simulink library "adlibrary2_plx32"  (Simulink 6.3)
undefined symbols (not defined in the file or in its folder): clock_ratio, program
libraries: xbsIndex_r4 x36, adlibrary2_plx32 x1

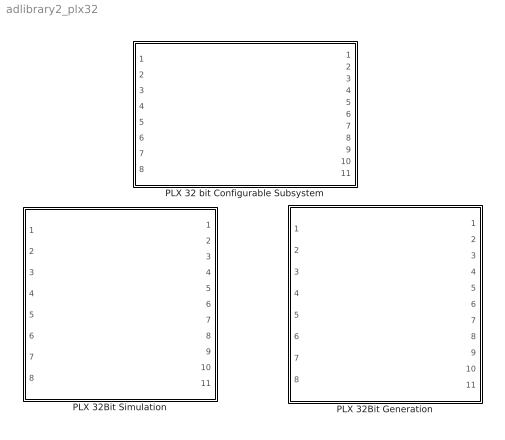
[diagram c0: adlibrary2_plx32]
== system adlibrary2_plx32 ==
  PLX 32 bit Configurable Subsystem : Subsystem  Tag=configX  BlockChoice=PLX 32Bit Simulation  mask{program=program, clock_ratio=clock_ratio}
      mask prompts: program "Local Bus Script Program"; clock_ratio "Clock Ratio"
  PLX 32Bit Generation : Subsystem
  PLX 32Bit Simulation : Subsystem  mask{program=program, clock_ratio=clock_ratio}
      mask prompts: program "Local Bus Script Program"; clock_ratio "Clock Ratio"

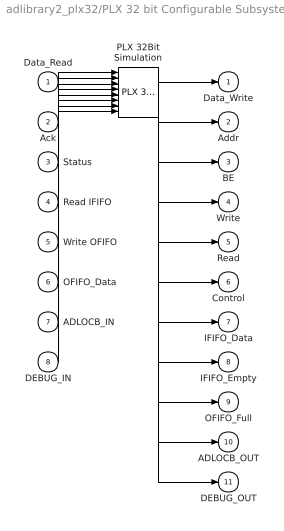
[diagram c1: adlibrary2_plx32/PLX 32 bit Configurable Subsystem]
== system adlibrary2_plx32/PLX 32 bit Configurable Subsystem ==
  Data_Read : Inport
  Ack : Inport  Port=2
  Status : Inport  Port=3
  Read IFIFO : Inport  Port=4
  Write OFIFO : Inport  Port=5
  OFIFO_Data : Inport  Port=6
  ADLOCB_IN : Inport  Port=7
  DEBUG_IN : Inport  Port=8
  PLX 32Bit Simulation : adlibrary2_plx32/PLX 32Bit Simulation  program=program  clock_ratio=clock_ratio
  Data_Write : Outport
  Addr : Outport  Port=2
  BE : Outport  Port=3
  Write : Outport  Port=4
  Read : Outport  Port=5
  Control : Outport  Port=6
  IFIFO_Data : Outport  Port=7
  IFIFO_Empty : Outport  Port=8
  OFIFO_Full : Outport  Port=9
  ADLOCB_OUT : Outport  Port=10
  DEBUG_OUT : Outport  Port=11
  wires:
  Data_Read/1 -> PLX 32Bit Simulation/1
  Ack/1 -> PLX 32Bit Simulation/2
  Status/1 -> PLX 32Bit Simulation/3
  Read IFIFO/1 -> PLX 32Bit Simulation/4
  Write OFIFO/1 -> PLX 32Bit Simulation/5
  OFIFO_Data/1 -> PLX 32Bit Simulation/6
  ADLOCB_IN/1 -> PLX 32Bit Simulation/7
  DEBUG_IN/1 -> PLX 32Bit Simulation/8
  PLX 32Bit Simulation/1 -> Data_Write/1
  PLX 32Bit Simulation/2 -> Addr/1
  PLX 32Bit Simulation/3 -> BE/1
  PLX 32Bit Simulation/4 -> Write/1
  PLX 32Bit Simulation/5 -> Read/1
  PLX 32Bit Simulation/6 -> Control/1
  PLX 32Bit Simulation/7 -> IFIFO_Data/1
  PLX 32Bit Simulation/8 -> IFIFO_Empty/1
  PLX 32Bit Simulation/9 -> OFIFO_Full/1
  PLX 32Bit Simulation/10 -> ADLOCB_OUT/1
  PLX 32Bit Simulation/11 -> DEBUG_OUT/1

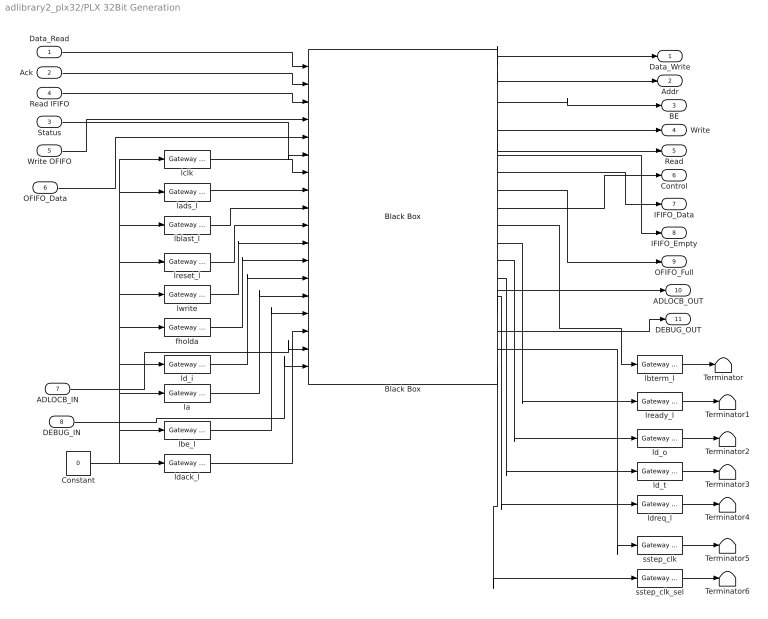
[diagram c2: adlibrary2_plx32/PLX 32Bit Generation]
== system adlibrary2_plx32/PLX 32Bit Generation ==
  Data_Read : Inport
  Ack : Inport  Port=2
  Status : Inport  Port=3
  Read IFIFO : Inport  Port=4
  Write OFIFO : Inport  Port=5
  OFIFO_Data : Inport  Port=6
  ADLOCB_IN : Inport  Port=7
  DEBUG_IN : Inport  Port=8
  Black Box : xbsIndex_r4/Black Box  init_code=lbif32_plx_config  sim_method=Inactive  block_type=blackbox2
  Constant : Constant  Value=0
  Terminator{,1..6} (7 alike) : Terminator
  fholda : xbsIndex_r4/Gateway In  arith_type=Boolean  n_bits=8  bin_pt=6  period=1  dbl_ovrd=off  timing_constraint=None  locs_specified=off  LOCs={}  block_type=gatewayin
  la : xbsIndex_r4/Gateway In  arith_type=Unsigned  n_bits=24  bin_pt=0  period=1  dbl_ovrd=off  timing_constraint=None  locs_specified=off  LOCs={}  block_type=gatewayin
  lads_l : xbsIndex_r4/Gateway In  arith_type=Boolean  n_bits=8  bin_pt=6  period=1  dbl_ovrd=off  timing_constraint=None  locs_specified=off  LOCs={}  block_type=gatewayin
  lbe_l : xbsIndex_r4/Gateway In  arith_type=Unsigned  n_bits=4  bin_pt=0  period=1  dbl_ovrd=off  timing_constraint=None  locs_specified=off  LOCs={}  block_type=gatewayin
  lblast_l : xbsIndex_r4/Gateway In  arith_type=Boolean  n_bits=8  bin_pt=6  period=1  dbl_ovrd=off  timing_constraint=None  locs_specified=off  LOCs={}  block_type=gatewayin
  lbterm_l : xbsIndex_r4/Gateway Out  hdl_port=on  timing_constraint=None  locs_specified=off  LOCs={}  block_type=gatewayout
  lclk : xbsIndex_r4/Gateway In  arith_type=Boolean  n_bits=8  bin_pt=6  period=1  dbl_ovrd=off  timing_constraint=None  locs_specified=off  LOCs={}  block_type=gatewayin
  ld_i : xbsIndex_r4/Gateway In  arith_type=Unsigned  n_bits=32  bin_pt=0  period=1  dbl_ovrd=off  timing_constraint=None  locs_specified=off  LOCs={}  block_type=gatewayin
  ld_o : xbsIndex_r4/Gateway Out  hdl_port=on  timing_constraint=None  locs_specified=off  LOCs={}  block_type=gatewayout
  ld_t : xbsIndex_r4/Gateway Out  hdl_port=on  timing_constraint=None  locs_specified=off  LOCs={}  block_type=gatewayout
  ldack_l : xbsIndex_r4/Gateway In  arith_type=Unsigned  n_bits=2  bin_pt=0  period=1  dbl_ovrd=off  timing_constraint=None  locs_specified=off  LOCs={}  block_type=gatewayin
  ldreq_l : xbsIndex_r4/Gateway Out  hdl_port=on  timing_constraint=None  locs_specified=off  LOCs={}  block_type=gatewayout
  lready_l : xbsIndex_r4/Gateway Out  hdl_port=on  timing_constraint=None  locs_specified=off  LOCs={}  block_type=gatewayout
  lreset_l : xbsIndex_r4/Gateway In  arith_type=Boolean  n_bits=8  bin_pt=6  period=1  dbl_ovrd=off  timing_constraint=None  locs_specified=off  LOCs={}  block_type=gatewayin
  lwrite : xbsIndex_r4/Gateway In  arith_type=Boolean  n_bits=8  bin_pt=6  period=1  dbl_ovrd=off  timing_constraint=None  locs_specified=off  LOCs={}  block_type=gatewayin
  sstep_clk : xbsIndex_r4/Gateway Out  hdl_port=on  timing_constraint=None  locs_specified=off  LOCs={}  block_type=gatewayout
  sstep_clk_sel : xbsIndex_r4/Gateway Out  hdl_port=on  timing_constraint=None  locs_specified=off  LOCs={}  block_type=gatewayout
  Data_Write : Outport
  Addr : Outport  Port=2
  BE : Outport  Port=3
  Write : Outport  Port=4
  Read : Outport  Port=5
  Control : Outport  Port=6
  IFIFO_Data : Outport  Port=7
  IFIFO_Empty : Outport  Port=8
  OFIFO_Full : Outport  Port=9
  ADLOCB_OUT : Outport  Port=10
  DEBUG_OUT : Outport  Port=11
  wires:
  Data_Read/1 -> Black Box/1
  Write OFIFO/1 -> Black Box/4
  OFIFO_Data/1 -> Black Box/5
  lclk/1 -> Black Box/7
  lblast_l/1 -> Black Box/9
  lreset_l/1 -> Black Box/10
  lwrite/1 -> Black Box/11
  fholda/1 -> Black Box/12
  ld_i/1 -> Black Box/13
  la/1 -> Black Box/14
  lbe_l/1 -> Black Box/15
  ldack_l/1 -> Black Box/16
  Constant/1 -> ldack_l/1, lclk/1, lads_l/1, lblast_l/1, lreset_l/1, lwrite/1, fholda/1, ld_i/1, la/1, lbe_l/1
  lbterm_l/1 -> Terminator/1
  lready_l/1 -> Terminator1/1
  ld_o/1 -> Terminator2/1
  ld_t/1 -> Terminator3/1
  ldreq_l/1 -> Terminator4/1
  Black Box/1 -> Data_Write/1
  Black Box/2 -> Addr/1
  Black Box/3 -> BE/1
  Black Box/4 -> Write/1
  Black Box/5 -> Read/1
  Black Box/7 -> IFIFO_Data/1
  Black Box/8 -> OFIFO_Full/1
  Black Box/6 -> IFIFO_Empty/1
  Black Box/9 -> Control/1
  Black Box/10 -> lbterm_l/1
  Black Box/11 -> lready_l/1
  Black Box/12 -> ld_o/1
  Black Box/13 -> ld_t/1
  Black Box/14 -> ldreq_l/1
  Ack/1 -> Black Box/2
  Read IFIFO/1 -> Black Box/3
  lads_l/1 -> Black Box/8
  Status/1 -> Black Box/6
  ADLOCB_IN/1 -> Black Box/17
  Black Box/15 -> ADLOCB_OUT/1
  sstep_clk/1 -> Terminator5/1
  sstep_clk_sel/1 -> Terminator6/1
  Black Box/17 -> sstep_clk/1
  Black Box/18 -> sstep_clk_sel/1
  Black Box/16 -> DEBUG_OUT/1
  DEBUG_IN/1 -> Black Box/18

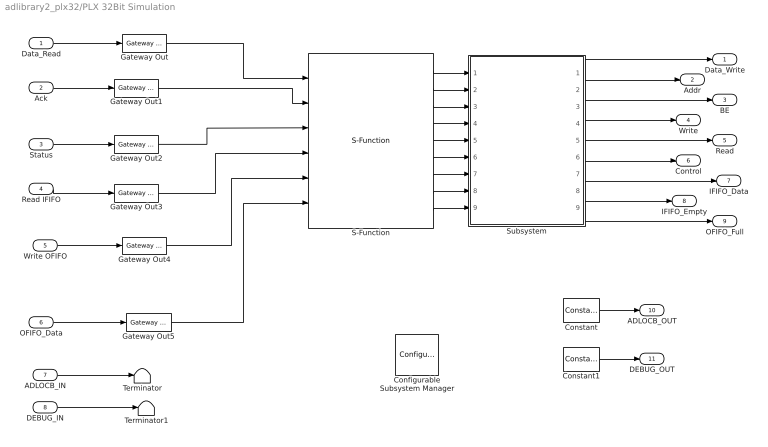
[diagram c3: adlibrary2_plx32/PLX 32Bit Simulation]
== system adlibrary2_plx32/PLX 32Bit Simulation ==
  Data_Read : Inport
  Ack : Inport  Port=2
  Status : Inport  Port=3
  Read IFIFO : Inport  Port=4
  Write OFIFO : Inport  Port=5
  OFIFO_Data : Inport  Port=6
  ADLOCB_IN : Inport  Port=7
  DEBUG_IN : Inport  Port=8
  Configurable Subsystem Manager : xbsIndex_r4/Configurable Subsystem Manager  Tag=xcfgMgr  block_type=configsubsys
  Constant : xbsIndex_r4/Constant  arith_type=Unsigned  const=0  n_bits=34  bin_pt=0  explicit_period=on  period=1  equ=P=C  opselect=C  inp2=PCIN>>17  opr=+  inp1=P  carry=CIN  dbl_ovrd=off  block_type=constant
  Constant1 : xbsIndex_r4/Constant  arith_type=Unsigned  const=0  n_bits=40  bin_pt=0  explicit_period=on  period=1  equ=P=C  opselect=C  inp2=PCIN>>17  opr=+  inp1=P  carry=CIN  dbl_ovrd=off  block_type=constant
  Gateway Out{,1..5} (6 alike) : xbsIndex_r4/Gateway Out  hdl_port=off  timing_constraint=None  locs_specified=off  LOCs={}  block_type=gatewayout
  S-Function : S-Function  FunctionName=lbif_plx32  Parameters=program,clock_ratio
  Subsystem : Subsystem
  Terminator : Terminator
  Terminator1 : Terminator
  Data_Write : Outport
  Addr : Outport  Port=2
  BE : Outport  Port=3
  Write : Outport  Port=4
  Read : Outport  Port=5
  Control : Outport  Port=6
  IFIFO_Data : Outport  Port=7
  IFIFO_Empty : Outport  Port=8
  OFIFO_Full : Outport  Port=9
  ADLOCB_OUT : Outport  Port=10
  DEBUG_OUT : Outport  Port=11
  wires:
  Subsystem/2(Out2) -> Addr/1
  Subsystem/1(Out1) -> Data_Write/1
  S-Function/2 -> Subsystem/2(In2)
  S-Function/1 -> Subsystem/1(In1)
  Gateway Out5/1 -> S-Function/6
  Gateway Out4/1 -> S-Function/5
  Gateway Out3/1 -> S-Function/4
  Gateway Out2/1 -> S-Function/3
  Gateway Out1/1 -> S-Function/2
  Gateway Out/1 -> S-Function/1
  OFIFO_Data/1 -> Gateway Out5/1
  Write OFIFO/1 -> Gateway Out4/1
  Read IFIFO/1 -> Gateway Out3/1
  Status/1 -> Gateway Out2/1
  Ack/1 -> Gateway Out1/1
  Data_Read/1 -> Gateway Out/1
  S-Function/3 -> Subsystem/3(In9)
  Subsystem/3(Out9) -> BE/1
  S-Function/4 -> Subsystem/4(In3)
  S-Function/5 -> Subsystem/5(In4)
  S-Function/6 -> Subsystem/6(In5)
  S-Function/7 -> Subsystem/7(In6)
  S-Function/8 -> Subsystem/8(In7)
  S-Function/9 -> Subsystem/9(In8)
  Subsystem/4(Out3) -> Write/1
  Subsystem/5(Out4) -> Read/1
  Subsystem/6(Out5) -> Control/1
  Subsystem/7(Out6) -> IFIFO_Data/1
  Subsystem/8(Out7) -> IFIFO_Empty/1
  Subsystem/9(Out8) -> OFIFO_Full/1
  ADLOCB_IN/1 -> Terminator/1
  Constant/1 -> ADLOCB_OUT/1
  DEBUG_IN/1 -> Terminator1/1
  Constant1/1 -> DEBUG_OUT/1

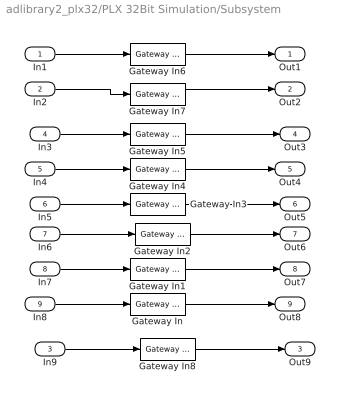
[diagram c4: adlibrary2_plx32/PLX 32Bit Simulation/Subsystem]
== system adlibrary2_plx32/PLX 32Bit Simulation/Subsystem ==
  In1 : Inport
  In2 : Inport  Port=2
  In9 : Inport  Port=3
  In3 : Inport  Port=4
  In4 : Inport  Port=5
  In5 : Inport  Port=6
  In6 : Inport  Port=7
  In7 : Inport  Port=8
  In8 : Inport  Port=9
  Gateway In{,1,4..5} (4 alike) : xbsIndex_r4/Gateway In  arith_type=Boolean  n_bits=8  bin_pt=6  period=1  dbl_ovrd=off  timing_constraint=None  locs_specified=off  LOCs={}  block_type=gatewayin
  Gateway In2 : xbsIndex_r4/Gateway In  arith_type=Unsigned  n_bits=32  bin_pt=0  period=1  dbl_ovrd=off  timing_constraint=None  locs_specified=off  LOCs={}  block_type=gatewayin
  Gateway In3 : xbsIndex_r4/Gateway In  arith_type=Unsigned  n_bits=32  bin_pt=0  period=1  dbl_ovrd=off  timing_constraint=None  locs_specified=off  LOCs={}  block_type=gatewayin
  Gateway In6 : xbsIndex_r4/Gateway In  arith_type=Unsigned  n_bits=32  bin_pt=0  period=1  dbl_ovrd=off  timing_constraint=None  locs_specified=off  LOCs={}  block_type=gatewayin
  Gateway In7 : xbsIndex_r4/Gateway In  arith_type=Unsigned  n_bits=16  bin_pt=0  period=1  dbl_ovrd=off  timing_constraint=None  locs_specified=off  LOCs={}  block_type=gatewayin
  Gateway In8 : xbsIndex_r4/Gateway In  arith_type=Unsigned  n_bits=4  bin_pt=0  period=1  dbl_ovrd=off  timing_constraint=None  locs_specified=off  LOCs={}  block_type=gatewayin
  Out1 : Outport
  Out2 : Outport  Port=2
  Out9 : Outport  Port=3
  Out3 : Outport  Port=4
  Out4 : Outport  Port=5
  Out5 : Outport  Port=6
  Out6 : Outport  Port=7
  Out7 : Outport  Port=8
  Out8 : Outport  Port=9
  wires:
  Gateway In8/1 -> Out9/1
  In9/1 -> Gateway In8/1
  Gateway In6/1 -> Out1/1
  Gateway In7/1 -> Out2/1
  Gateway In5/1 -> Out3/1
  Gateway In4/1 -> Out4/1
  Gateway In3/1 -> Out5/1
  Gateway In2/1 -> Out6/1
  Gateway In1/1 -> Out7/1
  Gateway In/1 -> Out8/1
  In8/1 -> Gateway In/1
  In7/1 -> Gateway In1/1
  In6/1 -> Gateway In2/1
  In5/1 -> Gateway In3/1
  In4/1 -> Gateway In4/1
  In3/1 -> Gateway In5/1
  In2/1 -> Gateway In7/1
  In1/1 -> Gateway In6/1
